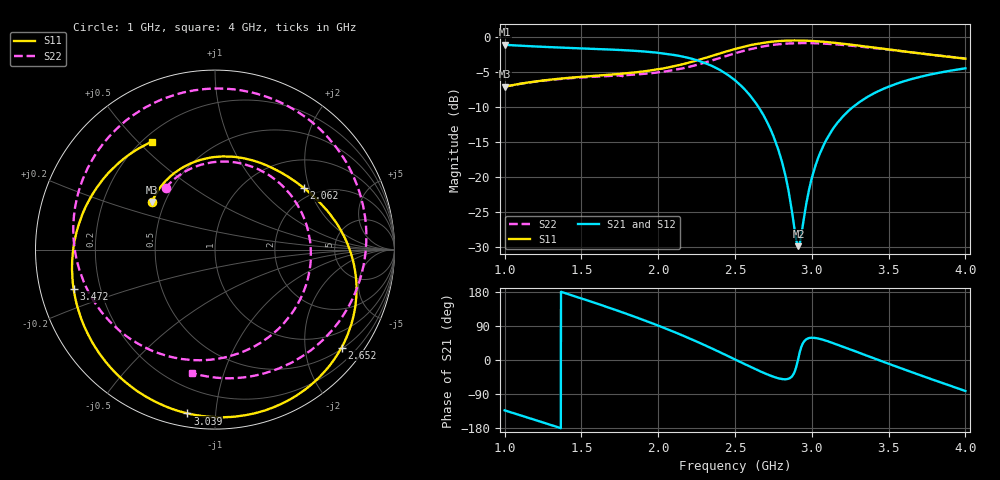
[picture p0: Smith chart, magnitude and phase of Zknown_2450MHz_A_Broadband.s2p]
!Agilent Technologies,N5242A,MY49421279,A.09.90.21
!Agilent N5242A: A.09.90.21
!Date: Monday, January 30, 2023
!Caliblation kit: 85033D 3.5mm Calibration Kit
!DUT Connector Gender Port1: male
!DUT Connector Gender Port2: female
!S2P File: Measurements: S11, S21, S12, S22:
# Hz S  dB  R 50
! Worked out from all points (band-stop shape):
!   3001 points, 1 GHz to 4 GHz, reference 50 ohm
!   highest |S21| = -1.17 dB at 1.001 GHz (marker M1); lowest = -29.8 dB at 2.913 GHz (marker M2)
!   |S21| within 3 dB of the highest: start of sweep to 2.349 GHz
!   lowest |S11| = -7.1 dB at 1 GHz (marker M3), VSWR 2.57, Z = 21.2 + j14 ohm
!   |S11| at or under -10 dB: nowhere
!   |S22| runs from -7.1 to -0.9 dB; largest |S21 - S12| = 0.014
!   S11 on the Smith chart (normalised r, x): 1 GHz: 0.42, +0.28; 2.062 GHz: 1.71, +1.84; 2.652 GHz: 0.53, -2.83; 3.039 GHz: 0.07, -0.84; 3.472 GHz: 0.10, -0.13; 4 GHz: 0.24, +0.55
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1e9  -7.12 143.0  -1.17 -132.9  -1.18 -132.8  -7.13 128.8
1.001e9  -7.12 142.8  -1.17 -133.0  -1.18 -132.9  -7.13 128.7
1.259e9  -6.23 113.9  -1.47 -166.0  -1.48 -165.9  -6.26 91.8
1.5e9  -5.72 88.5  -1.68 162.5  -1.69 162.6  -5.82 54.8
1.783e9  -5.24 60.6  -1.95 123.4  -1.94 123.6  -5.48 5.1
2e9  -4.65 40.5  -2.30 90.7  -2.29 90.9  -5.09 -40.3
2.062e9  -4.40 34.7  -2.47 80.8  -2.45 80.9  -4.90 -54.6
2.187e9  -3.78 22.5  -2.98 59.8  -2.95 59.9  -4.38 -85.5
2.292e9  -3.13 11.3  -3.66 41.1  -3.62 41.0  -3.78 -113.0
2.392e9  -2.46 -0.6  -4.63 22.4  -4.60 22.3  -3.11 -140.1
2.5e9  -1.76 -15.1  -6.22 1.5  -6.21 1.2  -2.38 -169.7
2.577e9  -1.33 -26.3  -7.84 -13.5  -7.84 -13.8  -1.91 169.5
2.652e9  -1.00 -37.8  -9.99 -27.7  -10.01 -28.0  -1.53 149.6
2.797e9  -0.62 -60.8  -17.13 -49.6  -17.18 -49.9  -1.06 113.0
2.913e9  -0.55 -79.5  -29.81 5.8  -29.88 5.7  -0.93 86.1
3e9  -0.62 -93.4  -20.15 58.7  -20.21 58.8  -0.94 67.2
3.039e9  -0.67 -99.5  -17.40 57.0  -17.47 57.0  -0.96 59.1
3.246e9  -1.13 -131.3  -10.43 28.7  -10.49 29.0  -1.28 19.1
3.472e9  -1.75 -164.5  -7.38 -5.7  -7.40 -5.2  -1.80 -19.8
3.5e9  -1.83 -168.5  -7.13 -9.9  -7.14 -9.4  -1.86 -24.4
3.743e9  -2.49 156.7  -5.53 -45.4  -5.51 -45.0  -2.49 -62.5
4e9  -3.14 120.3  -4.51 -81.8  -4.47 -81.5  -3.11 -100.4
